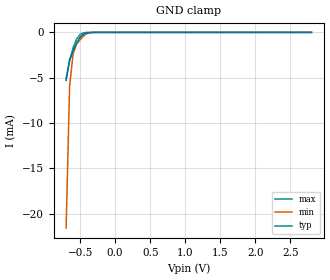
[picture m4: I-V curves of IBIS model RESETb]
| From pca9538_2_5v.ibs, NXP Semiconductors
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[Model]   RESETb
Model_type Input
Vinh=1.5
Vinl=0.75
C_comp   1.73p   1.7p   1.78p
[Temperature Range] 27   85   -40
[Voltage Range]   2.5   2.2   2.8
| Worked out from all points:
|   GND clamp passes 1 mA (typ) near -0.54 V on its own axis
[GND Clamp]
-700mV    -5.302mA   -21.58mA   -5.122mA
-650mV    -2.995mA   -5.963mA   -3.206mA
-600mV    -2.04mA    -2.358mA   -1.687mA
-550mV    -1.169mA   -1.297mA   -720.1uA
-500mV    -525.2uA   -816.9uA   -228.9uA
-450mV    -185.2uA   -388.2uA   -49.68uA
-400mV    -48.21uA   -135uA     -7.763uA
-350mV    -9.525uA   -35.75uA   -921.4nA
-250mV    -208.1nA   -1.277uA   -8.827nA
2.8V      51pA       210.6pA    36.58pA
